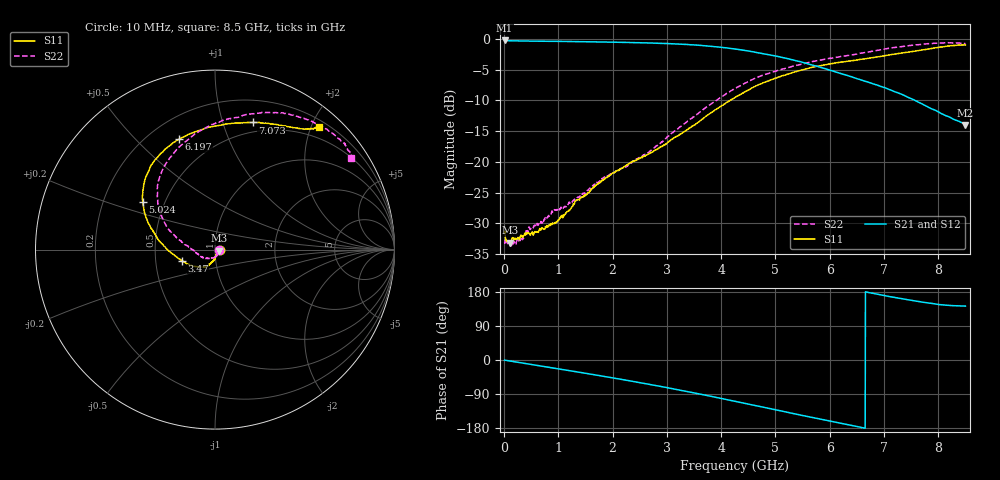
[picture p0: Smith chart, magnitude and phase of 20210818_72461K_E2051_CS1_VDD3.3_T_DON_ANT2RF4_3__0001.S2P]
!Agilent Technologies,E5071C,MY46417908,A.11.23
!Date: Wed Aug 18 14:33:47 2021
!Data & Calibration Information:
!Freq	S11:SOLT2(ON)	S21:SOLT2(ON)	S12:SOLT2(ON)	S22:SOLT2(ON)
!PortZ  Port1:50+j0  Port2:50+j0
!Above PortZ is port z conversion or system Z0 setting when saving the data.
!When reading, reference impedance value at option line is always used.
# Hz S dB R 50
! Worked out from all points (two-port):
!   1601 points, 10 MHz to 8.5 GHz, reference 50 ohm
!   highest |S21| = -0.24 dB at 10 MHz (marker M1); lowest = -14.0 dB at 8.5 GHz (marker M2)
!   |S21| within 3 dB of the highest: start of sweep to 5.246 GHz
!   lowest |S11| = -33.2 dB at 110.8 MHz (marker M3), VSWR 1.04, Z = 52.1 - j0.653 ohm
!   |S11| at or under -10 dB: start of sweep to 4.162 GHz
!   |S22| runs from -33.7 to -0.6 dB; largest |S21 - S12| = 0.0028
!   S11 on the Smith chart (normalised r, x): 10 MHz: 1.05, +0.00; 3.47 GHz: 0.68, -0.09; 5.024 GHz: 0.38, +0.26; 6.197 GHz: 0.32, +0.67; 7.073 GHz: 0.40, +1.26; 8.5 GHz: 0.31, +2.13
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1e7  -31.54 0.4  -0.24 -0.4  -0.24 -0.4  -33.02 -9.0
1.108188e8  -33.16 -16.6  -0.29 -2.8  -0.29 -2.7  -33.42 -21.4
3.336812e8  -32.02 -32.5  -0.33 -7.9  -0.32 -7.9  -32.59 -50.3
4.451125e8  -31.53 -45.6  -0.34 -10.5  -0.33 -10.5  -31.09 -56.5
9.439e8  -29.85 -80.3  -0.39 -21.9  -0.39 -22.0  -27.81 -81.6
1.426769e9  -25.82 -91.5  -0.44 -33.3  -0.44 -33.3  -25.33 -118.4
1.973312e9  -22.06 -107.2  -0.52 -46.5  -0.52 -46.5  -21.90 -145.6
2.843538e9  -17.78 -131.8  -0.70 -68.7  -0.70 -68.7  -17.16 176.8
3.469675e9  -14.19 -161.7  -0.96 -85.9  -0.96 -85.9  -12.85 162.2
3.904788e9  -11.49 179.7  -1.27 -98.6  -1.26 -98.5  -10.03 152.3
4.255e9  -9.53 167.6  -1.63 -109.1  -1.63 -109.1  -8.07 142.8
4.63705e9  -7.65 156.2  -2.18 -120.6  -2.18 -120.6  -6.33 131.6
5.024406e9  -6.30 146.4  -2.81 -132.0  -2.83 -132.1  -5.18 119.8
5.671769e9  -4.62 127.5  -4.24 -151.4  -4.26 -151.5  -3.69 99.9
6.197088e9  -3.79 108.1  -5.61 -166.5  -5.61 -166.7  -2.86 87.0
6.584444e9  -3.31 92.4  -6.68 -177.9  -6.67 -178.0  -2.30 77.7
7.072619e9  -2.63 73.5  -8.13 168.2  -8.15 168.1  -1.55 65.7
7.088538e9  -2.60 73.0  -8.19 167.7  -8.21 167.6  -1.53 65.3
7.528956e9  -2.03 60.4  -9.80 156.8  -9.80 156.7  -1.01 54.3
7.895088e9  -1.53 53.1  -11.42 149.0  -11.40 148.9  -0.73 45.0
8.128562e9  -1.21 50.8  -12.43 145.0  -12.40 145.0  -0.61 39.7
8.5e9  -0.97 49.6  -13.97 142.3  -13.94 142.1  -0.77 33.9
